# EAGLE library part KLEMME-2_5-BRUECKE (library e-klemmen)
Klemme 5-pol. mit Brückenhinweis
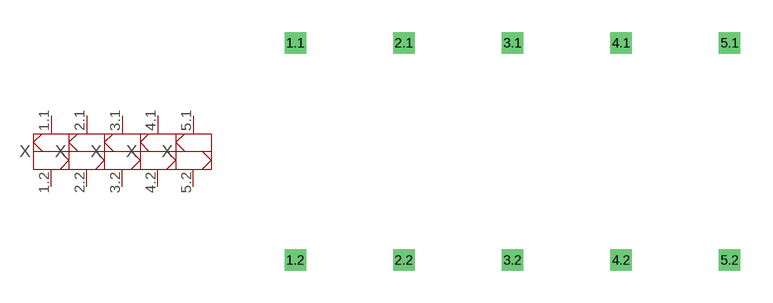
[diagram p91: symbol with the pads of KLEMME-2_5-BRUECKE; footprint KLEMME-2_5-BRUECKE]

Designator prefix X; gates 1=KLEMME-2_1-BRUECKE 2=KLEMME-2_2-BRUECKE 3=KLEMME-2_3-BRUECKE 4=KLEMME-2_4-BRUECKE 5=KLEMME-2_5-BRUECKE

## KLEMME-2_5-BRUECKE  [KLEMME-2_5-BRUECKE]
1.1  1:1  pas
1.2  1:2  pas
2.1  2:1  pas
2.2  2:2  pas
3.1  3:1  pas
3.2  3:2  pas
4.1  4:1  pas
4.2  4:2  pas
5.1  5:1  pas
5.2  5:2  pas

## Footprint KLEMME-2_5-BRUECKE (pad centres in mm)
Dummy
drill 0.5 pad 1 square: 1.1 0,5.08; 1.2 0,-5.08; 2.1 5.08,5.08; 2.2 5.08,-5.08; 3.1 10.16,5.08; 3.2 10.16,-5.08; 4.1 15.24,5.08; 4.2 15.24,-5.08; 5.1 20.32,5.08; 5.2 20.32,-5.08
